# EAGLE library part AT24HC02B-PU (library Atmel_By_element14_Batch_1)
Two-wire Serial EEPROM
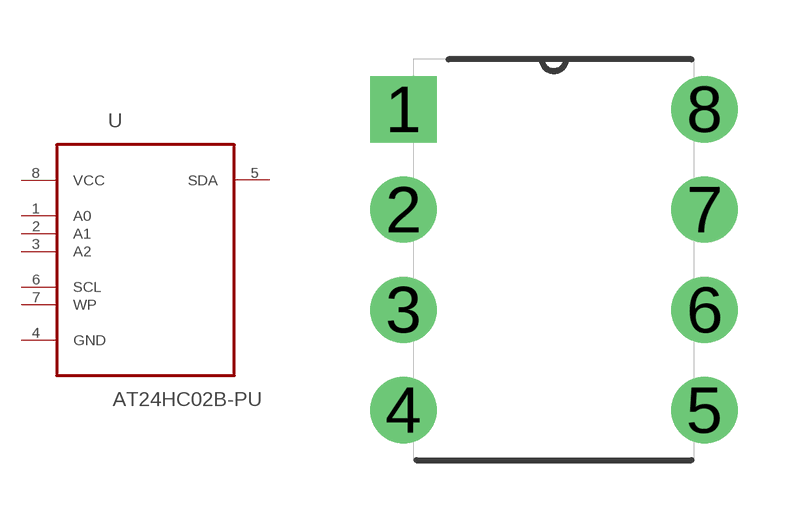
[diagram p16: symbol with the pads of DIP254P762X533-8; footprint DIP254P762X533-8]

Designator prefix U

## AT24HC02B-PU (MPN: AT24HC02B-PU; OC_FARNELL: 1362640; OC_NEWARK: 50M3331; PACKAGE: PDIP-8; SUPPLIER: Atmel)  [DIP254P762X533-8]
1  A0  in
2  A1  in
3  A2  in
4  GND  pas
5  SDA
6  SCL  in
7  WP  in
8  VCC  pwr

## Footprint DIP254P762X533-8 (pad centres in mm)
drill 1.118 square: 1 -7.62,7.62
drill 1.118: 2 -7.62,5.08; 3 -7.62,2.54; 4 -7.62,0; 5 0,0; 6 0,2.54; 7 0,5.08; 8 0,7.62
